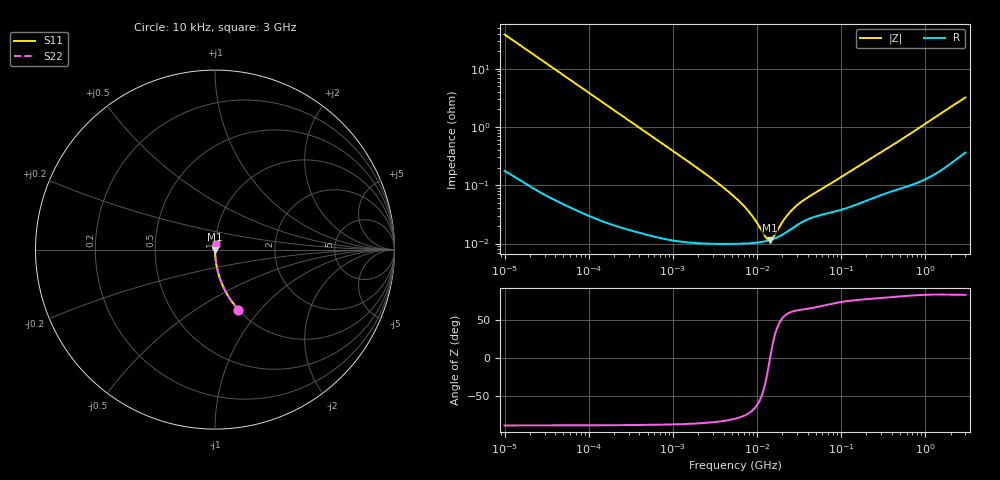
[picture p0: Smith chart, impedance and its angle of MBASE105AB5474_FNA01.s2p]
! MBASE105AB5474_FNA01  S-PARAMETER MODEL  ( Standard Model )
! Model Generated by TAIYO YUDEN Corporation (http://www.ty-top.com)
! Version 1.0
! TAIYO YUDEN Control No. 220601
! Copyright(c) 2013 TAIYO YUDEN CO.,LTD. All Rights Reserved.
! Product Description (link to TY-COMPAS)
! https://ds.yuden.co.jp/TYCOMPAS/or/detail?pn=MBASE105AB5474KFNA01&u=M
! Products Name : Multilayer Ceramic Capacitors
! Characteristics :
!  Capacitance : 0.47 [uF] , Rated Voltage : 16 [V] , TCC : X5R
!  Case Size : 1.0 x 0.5 / 0.039 x 0.02 [mm/inch] , Thickness : 0.5 / 0.02 [mm/inch]
!  (Conditions: Temperature = 25 [degC] , DC Bias Voltage = 0 [V])
! External Node Assignments :
!  1  o---| |---o  2
! GND o---------o GND
! Frequency Range : 10kHz  -  3GHz  [ 401 STEP ]
# MHZ S RI R 50
! Freq[MHz].  S11 Real  S11 Imag  S21 Real  S21 Imag  S12 Real  S12 Imag  S22 Real  S22 Imag
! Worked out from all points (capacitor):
!   401 points, 10 kHz to 3 GHz, reference 50 ohm
!   read as one part in series: C = 413 nF near 10.65 kHz
!   lowest |Z| = 11.5 mohm at 14.1 MHz (marker M1)
!   series resonance near 14.31 MHz, so ESL is about 300 pH
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0.01  0.1303 -0.3344  0.8697 0.3344  0.8697 0.3344  0.1303 -0.3344
0.016047  0.0556 -0.2268  0.9444 0.2268  0.9444 0.2268  0.0556 -0.2268
0.027426  0.0201 -0.1379  0.9799 0.1379  0.9799 0.1379  0.0201 -0.1379
0.045421  0.0077 -0.0845  0.9923 0.0845  0.9923 0.0845  0.0077 -0.0845
0.082683  0.00253 -0.0467  0.9975 0.0467  0.9975 0.0467  0.00253 -0.0467
0.199902  0.000583 -0.0194  0.9994 0.0194  0.9994 0.0194  0.000583 -0.0194
0.683653  0.000158 -0.0057  0.9998 0.0057  0.9998 0.0057  0.000158 -0.0057
2.652321  0.000102 -0.00143  0.9999 0.00143  0.9999 0.00143  0.000102 -0.00143
3.996065  9.94e-05 -0.000906  0.9999 0.000906  0.9999 0.000906  9.94e-05 -0.000906
5.477226  9.92e-05 -0.000613  0.9999 0.000613  0.9999 0.000613  9.92e-05 -0.000613
7.996027  0.000101 -0.000339  0.9999 0.000339  0.9999 0.000339  0.000101 -0.000339
9.6612  0.000103 -0.000222  0.9999 0.000222  0.9999 0.000222  0.000103 -0.000222
12.43293  0.000109 -7.8e-05  0.9999 7.8e-05  0.9999 7.8e-05  0.000109 -7.8e-05
13.24217  0.000111 -4.3e-05  0.9999 4.3e-05  0.9999 4.3e-05  0.000111 -4.3e-05
14.10408  0.000114 -8.1e-06  0.9999 8.1e-06  0.9999 8.1e-06  0.000114 -8.1e-06
15.50326  0.000119 4.41e-05  0.9999 -4.41e-05  0.9999 -4.41e-05  0.000119 4.41e-05
20.5901  0.000145 0.000201  0.9999 -0.000201  0.9999 -0.000201  0.000145 0.000201
25.67485  0.000179 0.000323  0.9998 -0.000323  0.9998 -0.000323  0.000179 0.000323
33.04079  0.000226 0.000457  0.9998 -0.000457  0.9998 -0.000457  0.000226 0.000457
45.28751  0.000279 0.000631  0.9997 -0.000631  0.9997 -0.000631  0.000279 0.000631
374.4521  0.000779 0.00445  0.9992 -0.00445  0.9992 -0.00445  0.000779 0.00445
3000  0.00463 0.0315  0.9954 -0.0315  0.9954 -0.0315  0.00463 0.0315
